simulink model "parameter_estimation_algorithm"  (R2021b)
settings: Solver=FixedStepDiscrete  StartTime=0.0  StopTime=10.0  RelTol=1e-3
InitFcn:
  | parameter_estimation_init;
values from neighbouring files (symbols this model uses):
  ADC_resolution = 12    [parameter_estimation_init.m]
  Ts = 1/PWM_frequency    (= 5e-05)    [parameter_estimation_init.m]
undefined symbols (not defined in the file or in its folder): bits, case, DiscIntNeverNeededParam, inverter
libraries: mcbcontrolslib x14, mcbpositiondecoderlib x3, simulink x2
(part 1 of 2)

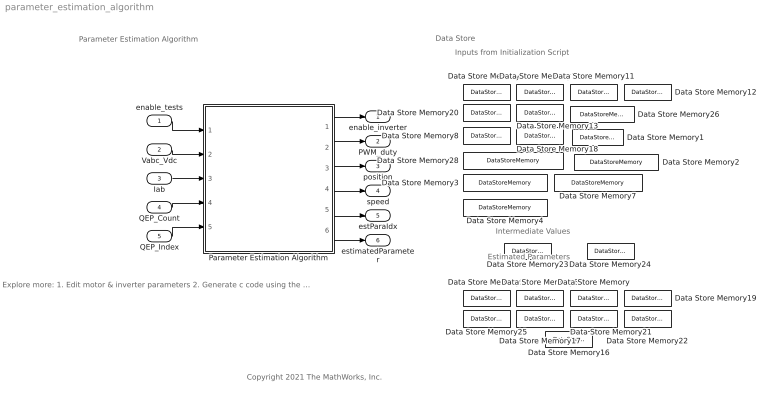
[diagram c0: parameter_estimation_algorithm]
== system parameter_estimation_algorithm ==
  note: Estimated Parameters
  note: Inputs from Initialization Script
  note: Data Store
  note: Intermediate Values
  note: Explore more: 1. Edit motor & inverter parameters 2. Generate c code using the 'Embedded Coder' app 3. Integrate generated code with driver code
  note: Parameter Estimation Algorithm
  note: Copyright 2021 The MathWorks, Inc.
  enable_tests : Inport  OutDataTypeStr=single
  Vabc_Vdc : Inport  Port=2  OutDataTypeStr=uint16
  Iab : Inport  Port=3  OutDataTypeStr=uint16
  QEP_Count : Inport  Port=4  OutDataTypeStr=uint16
  QEP_Index : Inport  Port=5  OutDataTypeStr=uint16
  Data Store Memory : DataStoreMemory  DataStoreName=Rs  ReadBeforeWriteMsg=warning  WriteAfterWriteMsg=warning  WriteAfterReadMsg=warning  ShowAdditionalParam=off  OutDataTypeStr=single
  Data Store Memory1 : DataStoreMemory  DataStoreName=testEnable  ReadBeforeWriteMsg=warning  WriteAfterWriteMsg=warning  WriteAfterReadMsg=warning  ShowAdditionalParam=off  OutDataTypeStr=single
  Data Store Memory10 : DataStoreMemory  DataStoreName=V_rated  ReadBeforeWriteMsg=warning  WriteAfterWriteMsg=warning  WriteAfterReadMsg=warning  InitialValue=motorParam.v_dc  ShowAdditionalParam=off  OutDataTypeStr=single
  Data Store Memory11 : DataStoreMemory  DataStoreName=speed_rated  ReadBeforeWriteMsg=warning  WriteAfterWriteMsg=warning  WriteAfterReadMsg=warning  InitialValue=motorParam.ratedSpeed  ShowAdditionalParam=off  OutDataTypeStr=single
  Data Store Memory12 : DataStoreMemory  DataStoreName=pole_pairs  ReadBeforeWriteMsg=warning  WriteAfterWriteMsg=warning  WriteAfterReadMsg=warning  InitialValue=motorParam.p  ShowAdditionalParam=off  OutDataTypeStr=single
  Data Store Memory13 : DataStoreMemory  DataStoreName=RsMeasTestTime  ReadBeforeWriteMsg=warning  WriteAfterWriteMsg=warning  WriteAfterReadMsg=warning  InitialValue=RsMeasTestTime  ShowAdditionalParam=off  OutDataTypeStr=single
  Data Store Memory16 : DataStoreMemory  DataStoreName=Ld  ReadBeforeWriteMsg=warning  WriteAfterWriteMsg=warning  WriteAfterReadMsg=warning  ShowAdditionalParam=off
  Data Store Memory17 : DataStoreMemory  DataStoreName=Lq  ReadBeforeWriteMsg=warning  WriteAfterWriteMsg=warning  WriteAfterReadMsg=warning  ShowAdditionalParam=off
  Data Store Memory18 : DataStoreMemory  DataStoreName=sigma  ReadBeforeWriteMsg=warning  WriteAfterWriteMsg=warning  WriteAfterReadMsg=warning  InitialValue=Ts * 1e6  ShowAdditionalParam=off  OutDataTypeStr=single
  Data Store Memory19 : DataStoreMemory  DataStoreName=Bemf  ReadBeforeWriteMsg=warning  WriteAfterWriteMsg=warning  WriteAfterReadMsg=warning  ShowAdditionalParam=off
  Data Store Memory2 : DataStoreMemory  DataStoreName=FrequencySweepMax  ReadBeforeWriteMsg=warning  WriteAfterWriteMsg=warning  WriteAfterReadMsg=warning  InitialValue=FrequencySweepMax  ShowAdditionalParam=off  OutDataTypeStr=single
  Data Store Memory20 : DataStoreMemory  DataStoreName=R_board  ReadBeforeWriteMsg=warning  WriteAfterWriteMsg=warning  WriteAfterReadMsg=warning  InitialValue=inverter.R_board  ShowAdditionalParam=off
  Data Store Memory21 : DataStoreMemory  DataStoreName=J  ReadBeforeWriteMsg=warning  WriteAfterWriteMsg=warning  WriteAfterReadMsg=warning  ShowAdditionalParam=off
  Data Store Memory22 : DataStoreMemory  DataStoreName=B  ReadBeforeWriteMsg=warning  WriteAfterWriteMsg=warning  WriteAfterReadMsg=warning  ShowAdditionalParam=off
  Data Store Memory23 : DataStoreMemory  DataStoreName=Kp_i  ReadBeforeWriteMsg=warning  WriteAfterWriteMsg=warning  WriteAfterReadMsg=warning  ShowAdditionalParam=off  OutDataTypeStr=single
  Data Store Memory24 : DataStoreMemory  DataStoreName=Ki_i  ReadBeforeWriteMsg=warning  WriteAfterWriteMsg=warning  WriteAfterReadMsg=warning  ShowAdditionalParam=off  OutDataTypeStr=single
  Data Store Memory25 : DataStoreMemory  DataStoreName=errorID  ReadBeforeWriteMsg=warning  WriteAfterWriteMsg=warning  WriteAfterReadMsg=warning  ShowAdditionalParam=off
  Data Store Memory26 : DataStoreMemory  DataStoreName=Position_offset  ReadBeforeWriteMsg=warning  WriteAfterWriteMsg=warning  WriteAfterReadMsg=warning  InitialValue=motorParam.PositionOffset  ShowAdditionalParam=off  OutDataTypeStr=single
  Data Store Memory28 : DataStoreMemory  DataStoreName=inverter_V_max  ReadBeforeWriteMsg=warning  WriteAfterWriteMsg=warning  WriteAfterReadMsg=warning  InitialValue=inverter.V_max  ShowAdditionalParam=off  OutDataTypeStr=single
  Data Store Memory3 : DataStoreMemory  DataStoreName=FrequencySweepMin  ReadBeforeWriteMsg=warning  WriteAfterWriteMsg=warning  WriteAfterReadMsg=warning  InitialValue=FrequencySweepMin  ShowAdditionalParam=off  OutDataTypeStr=single
  Data Store Memory4 : DataStoreMemory  DataStoreName=FrequencySweepStep  ReadBeforeWriteMsg=warning  WriteAfterWriteMsg=warning  WriteAfterReadMsg=warning  InitialValue=FrequencySweepStep  ShowAdditionalParam=off  OutDataTypeStr=single
  Data Store Memory5 : DataStoreMemory  DataStoreName=Ia_avg_cal  ReadBeforeWriteMsg=warning  WriteAfterWriteMsg=warning  WriteAfterReadMsg=warning  ShowAdditionalParam=off  OutDataTypeStr=single
  Data Store Memory6 : DataStoreMemory  DataStoreName=Ib_avg_cal  ReadBeforeWriteMsg=warning  WriteAfterWriteMsg=warning  WriteAfterReadMsg=warning  ShowAdditionalParam=off  OutDataTypeStr=single
  Data Store Memory7 : DataStoreMemory  DataStoreName=DaxisVoltageReference  ReadBeforeWriteMsg=warning  WriteAfterWriteMsg=warning  WriteAfterReadMsg=warning  InitialValue=DaxisVoltageReference  ShowAdditionalParam=off  OutDataTypeStr=single
  Data Store Memory8 : DataStoreMemory  DataStoreName=currentPU_RWV  ReadBeforeWriteMsg=warning  WriteAfterWriteMsg=warning  WriteAfterReadMsg=warning  InitialValue=inverter.I_max  ShowAdditionalParam=off  OutDataTypeStr=single
  Data Store Memory9 : DataStoreMemory  DataStoreName=I_rated  ReadBeforeWriteMsg=warning  WriteAfterWriteMsg=warning  WriteAfterReadMsg=warning  InitialValue=motorParam.nomCurrent  ShowAdditionalParam=off  OutDataTypeStr=single
  Parameter Estimation Algorithm : Subsystem
  enable_inverter : Outport
  PWM_duty : Outport  Port=2
  position : Outport  Port=3
  speed : Outport  Port=4
  estParaIdx : Outport  Port=5
  estimatedParameter : Outport  Port=6
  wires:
  QEP_Index/1 -> Parameter Estimation Algorithm/5(QEP_Index)
  Parameter Estimation Algorithm/2(PWM_duty) -> PWM_duty/1
  Vabc_Vdc/1 -> Parameter Estimation Algorithm/2(Vabc_Vdc)
  Iab/1 -> Parameter Estimation Algorithm/3(Iab)
  enable_tests/1 -> Parameter Estimation Algorithm/1(enable)
  QEP_Count/1 -> Parameter Estimation Algorithm/4(QEP_Count)
  Parameter Estimation Algorithm/1(enable_inverter) -> enable_inverter/1
  Parameter Estimation Algorithm/3(Position) -> position/1
  Parameter Estimation Algorithm/4(Speed) -> speed/1
  Parameter Estimation Algorithm/5(estParIdx) -> estParaIdx/1
  Parameter Estimation Algorithm/6(estimatedParameter) -> estimatedParameter/1

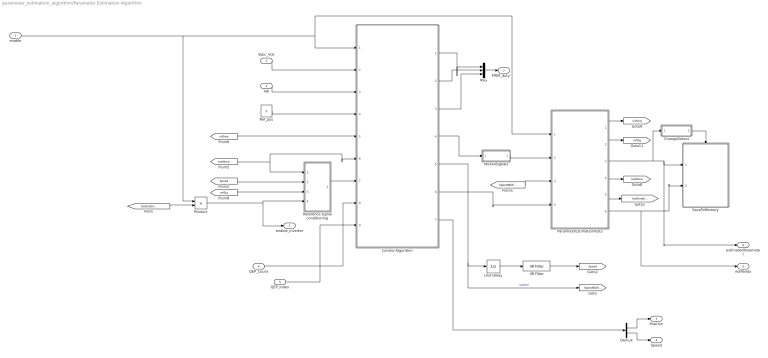
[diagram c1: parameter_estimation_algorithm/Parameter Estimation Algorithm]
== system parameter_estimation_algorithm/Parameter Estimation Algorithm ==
  enable : Inport
  Vabc_Vdc : Inport  Port=2  PortDimensions=4
  Iab : Inport  Port=3  PortDimensions=2
  QEP_Count : Inport  Port=4
  QEP_Index : Inport  Port=5
  ChangeDetect : Subsystem
  Control Algorithm : Subsystem
  Demux : Demux  Outputs=2
  IIR Filter : mcbcontrolslib/IIR Filter  VariantControl=Low Pass Filter  VariantSelect=Low-pass  Filter_constant=0.01  advancedSettings=off  Ts=50e-6  cutOff_freq=32.1525
  Mux : Mux  Inputs=3
  MuxAllSignals : Subsystem
  ParameterEstimationTests : Subsystem
  Product : Product  OutDataTypeStr=single
  Ref_pos : Constant  Value=0  OutDataTypeStr=single  SampleTime=-1
  Reference signal conditioning : Subsystem
  SaveToMemory : Subsystem
  Unit Delay : UnitDelay  SampleTime=-1  HasFrameUpgradeWarning=on
  enable_inverter : Outport
  PWM_duty : Outport  Port=2
  Position : Outport  Port=3
  Speed : Outport  Port=4
  estParIdx : Outport  Port=5
  estimatedParameter : Outport  Port=6
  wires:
  [testNum] -> Reference signal conditioning/1(TestNum), Control Algorithm/6(TestNum)
  [injFreq] -> Control Algorithm/5(Freq)
  Control Algorithm/4(Ia_Ib_ADC_count or VdId or VqIq or VaVb) -> MuxAllSignals/1(Sig)
  [Speed] -> Reference signal conditioning/2(ActSpeed)
  Control Algorithm/5(Speed) -> [SpeedWOfilter], Unit Delay/1  "speed"
  Reference signal conditioning/1(Out2) -> Control Algorithm/7(RefSignal)
  Control Algorithm/6(Vdc) -> ParameterEstimationTests/4(Vdc)
  ParameterEstimationTests/2(refSignalOut) -> [refSig]
  ParameterEstimationTests/1(injFreqOut) -> [injFreq]
  [refSig] -> Reference signal conditioning/3("RefSignal ")
  Product/1 -> enable_inverter/1, Reference signal conditioning/4(Running)
  ParameterEstimationTests/3(estimatedParameter) -> estimatedParameter/1, SaveToMemory/1(estimatedParameter), ChangeDetect/1(Sig)
  ChangeDetect/1(ChangeDet) -> SaveToMemory/Trigger
  ParameterEstimationTests/4(testNumOut) -> [testNum]
  MuxAllSignals/1(AllSig) -> ParameterEstimationTests/2(SignalPU)
  ParameterEstimationTests/6(estParIdx) -> estParIdx/1, SaveToMemory/2(estParIdx)
  ParameterEstimationTests/5(testEnableFromTrgt) -> [testEnableFromTrgt]
  [testEnableFromTrgt] -> Product/2
  Unit Delay/1 -> IIR Filter/1
  IIR Filter/1 -> [Speed]
  [SpeedWOfilter] -> ParameterEstimationTests/3(speed)
  Vabc_Vdc/1 -> Control Algorithm/2(Vabc_Vdc)
  Iab/1 -> Control Algorithm/3(IA/IB)
  Ref_pos/1 -> Control Algorithm/4(Ref_pos)
  Control Algorithm/1(PWM1) -> Mux/1
  Control Algorithm/2(PWM2) -> Mux/2
  Control Algorithm/3(PWM3) -> Mux/3
  QEP_Count/1 -> Control Algorithm/8(QEP_Count)
  QEP_Index/1 -> Control Algorithm/9(QEP_Index)
  enable/1 -> Product/1, ParameterEstimationTests/1(enable), Control Algorithm/1(enable)
  Mux/1 -> PWM_duty/1
  Control Algorithm/7(Pos/Speed) -> Demux/1
  Demux/1 -> Position/1
  Demux/2 -> Speed/1

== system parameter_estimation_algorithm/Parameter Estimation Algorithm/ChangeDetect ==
  Sig : Inport
  Equal : RelationalOperator  Operator=~=  OutDataTypeStr=boolean  RndMeth=Simplest
  Unit Delay : UnitDelay  SampleTime=-1  HasFrameUpgradeWarning=on
  ChangeDet : Outport
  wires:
  Equal/1 -> ChangeDet/1
  Sig/1 -> Equal/2, Unit Delay/1
  Unit Delay/1 -> Equal/1

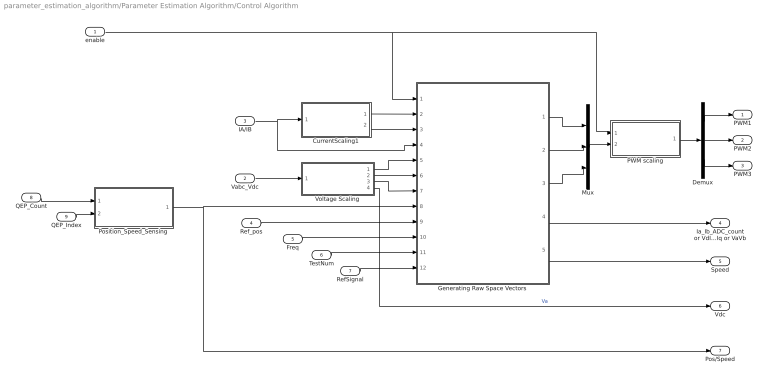
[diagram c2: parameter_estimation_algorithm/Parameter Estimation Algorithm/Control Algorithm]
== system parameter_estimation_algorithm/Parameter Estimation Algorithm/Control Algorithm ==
  enable : Inport
  Vabc_Vdc : Inport  Port=2
  IA/IB : Inport  Port=3
  Ref_pos : Inport  Port=4
  Freq : Inport  Port=5
  TestNum : Inport  Port=6
  RefSignal : Inport  Port=7
  QEP_Count : Inport  Port=8
  QEP_Index : Inport  Port=9
  CurrentScaling1 : Subsystem
  Demux : Demux  Outputs=3
  Generating Raw Space Vectors : Subsystem
  Mux : Mux  Inputs=3
  PWM scaling : Subsystem
  Position_Speed_Sensing : Subsystem
  Voltage Scaling : Subsystem
  PWM1 : Outport  VectorParamsAs1DForOutWhenUnconnected=off
  PWM2 : Outport  Port=2  VectorParamsAs1DForOutWhenUnconnected=off
  PWM3 : Outport  Port=3  VectorParamsAs1DForOutWhenUnconnected=off
  Ia_Ib_ADC_count or VdId or VqIq or VaVb : Outport  Port=4  OutDataTypeStr=single  VectorParamsAs1DForOutWhenUnconnected=off
  Speed : Outport  Port=5  OutDataTypeStr=single  VectorParamsAs1DForOutWhenUnconnected=off
  Vdc : Outport  Port=6  OutDataTypeStr=single  VectorParamsAs1DForOutWhenUnconnected=off
  Pos/Speed : Outport  Port=7
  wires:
  Demux/1 -> PWM1/1
  Demux/3 -> PWM3/1
  Demux/2 -> PWM2/1
  Vabc_Vdc/1 -> Voltage Scaling/1(Vabc)
  IA/IB/1 -> Generating Raw Space Vectors/4(IaIb_adc_counts), CurrentScaling1/1(IA/IB)
  Generating Raw Space Vectors/2(Tb) -> Mux/2
  Voltage Scaling/1(Vao) -> Generating Raw Space Vectors/5(Va0)
  Mux/1 -> PWM scaling/2(Ta/Tb/Tc)
  PWM scaling/1(PWM A/B/C) -> Demux/1
  CurrentScaling1/2(Ib) -> Generating Raw Space Vectors/3(Ib)
  CurrentScaling1/1(Ia) -> Generating Raw Space Vectors/2(Ia)
  Generating Raw Space Vectors/3(Tc) -> Mux/3
  Generating Raw Space Vectors/1(Ta) -> Mux/1
  Ref_pos/1 -> Generating Raw Space Vectors/9(Ref_posOL)
  Freq/1 -> Generating Raw Space Vectors/10(Freq)
  TestNum/1 -> Generating Raw Space Vectors/11(TestNum)
  RefSignal/1 -> Generating Raw Space Vectors/12(RefSignal)
  Generating Raw Space Vectors/4(Ia_Ib_ADC_count or VdId or VqIq or VaVb) -> Ia_Ib_ADC_count or VdId or VqIq or VaVb/1
  Generating Raw Space Vectors/5(Speed) -> Speed/1
  Voltage Scaling/2(Vbo) -> Generating Raw Space Vectors/6(Vb0)
  Voltage Scaling/3(Vco) -> Generating Raw Space Vectors/7(Vco)
  Position_Speed_Sensing/1(Pos/Speed) -> Pos/Speed/1, Generating Raw Space Vectors/8(Pos/Speed)
  Voltage Scaling/4(Vdc) -> Vdc/1  "Va"
  QEP_Count/1 -> Position_Speed_Sensing/1(QEP_Count)
  QEP_Index/1 -> Position_Speed_Sensing/2(QEP_Index)
  enable/1 -> PWM scaling/1(enable), Generating Raw Space Vectors/1(enable)

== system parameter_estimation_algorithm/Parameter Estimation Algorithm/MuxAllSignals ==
  Sig : Inport
  Demux : Demux  Outputs=2
  Demux1 : Demux  Outputs=2
  Demux2 : Demux  Outputs=2
  Mux : Mux  Inputs=6
  AllSig : Outport
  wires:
  Mux/1 -> AllSig/1
  Sig/1 -> Demux/1
  Demux/1 -> Mux/1
  Demux/2 -> Mux/2
  Demux1/2 -> Mux/4
  Demux1/1 -> Mux/3
  Demux2/1 -> Mux/5
  Demux2/2 -> Mux/6
  [VdId_32_Q17] -> Demux1/1
  [VqIq_32_Q17] -> Demux2/1

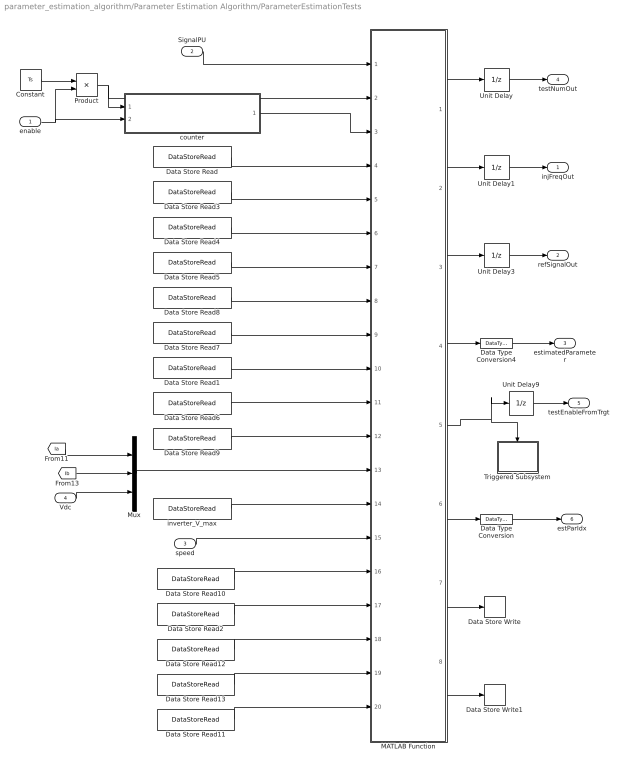
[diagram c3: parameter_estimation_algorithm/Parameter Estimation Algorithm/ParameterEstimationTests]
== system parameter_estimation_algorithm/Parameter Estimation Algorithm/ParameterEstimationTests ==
  enable : Inport
  SignalPU : Inport  Port=2
  speed : Inport  Port=3
  Vdc : Inport  Port=4
  Constant : Constant  Value=Ts  OutDataTypeStr=single  SampleTime=-1
  Data Store Read : DataStoreRead  DataStoreName=RsMeasTestTime  IndexOptions=Index vector (dialog)  Indices=1  OutputSizes=1
  Data Store Read1 : DataStoreRead  DataStoreName=V_rated  IndexOptions=Index vector (dialog)  Indices=1  OutputSizes=1
  Data Store Read10 : DataStoreRead  DataStoreName=speed_rated  IndexOptions=Index vector (dialog)  Indices=1  OutputSizes=1
  Data Store Read11 : DataStoreRead  DataStoreName=FrequencySweepStep  IndexOptions=Index vector (dialog)  Indices=1  OutputSizes=1
  Data Store Read12 : DataStoreRead  DataStoreName=FrequencySweepMin  IndexOptions=Index vector (dialog)  Indices=1  OutputSizes=1
  Data Store Read13 : DataStoreRead  DataStoreName=FrequencySweepMax  IndexOptions=Index vector (dialog)  Indices=1  OutputSizes=1
  Data Store Read2 : DataStoreRead  DataStoreName=DaxisVoltageReference  IndexOptions=Index vector (dialog)  Indices=1  OutputSizes=1
  Data Store Read3 : DataStoreRead  DataStoreName=I_rated  IndexOptions=Index vector (dialog)  Indices=1  OutputSizes=1
  Data Store Read4 : DataStoreRead  DataStoreName=pole_pairs  IndexOptions=Index vector (dialog)  Indices=1  OutputSizes=1
  Data Store Read5 : DataStoreRead  DataStoreName=Rs  IndexOptions=Index vector (dialog)  Indices=1  OutputSizes=1
  Data Store Read6 : DataStoreRead  DataStoreName=currentPU_RWV  IndexOptions=Index vector (dialog)  Indices=1  OutputSizes=1
  Data Store Read7 : DataStoreRead  DataStoreName=R_board  IndexOptions=Index vector (dialog)  Indices=1  OutputSizes=1
  Data Store Read8 : DataStoreRead  DataStoreName=Ld  IndexOptions=Index vector (dialog)  Indices=1  OutputSizes=1
  Data Store Read9 : DataStoreRead  DataStoreName=sigma  IndexOptions=Index vector (dialog)  Indices=1  OutputSizes=1
  Data Store Write : DataStoreWrite  DataStoreName=Kp_i  IndexOptions=Index vector (dialog)  Indices=1  OutputSizes=1
  Data Store Write1 : DataStoreWrite  DataStoreName=Ki_i  IndexOptions=Index vector (dialog)  Indices=1  OutputSizes=1
  Data Type Conversion : DataTypeConversion  OutDataTypeStr=uint32  RndMeth=Simplest
  Data Type Conversion4 : DataTypeConversion  OutDataTypeStr=single  RndMeth=Simplest
  MATLAB Function : MATLAB Function  TreatAsAtomicUnit=on
  Mux : Mux  Inputs=3
  Product : Product  OutDataTypeStr=single
  Triggered Subsystem : Subsystem  TreatAsAtomicUnit=on
  Unit Delay : UnitDelay  SampleTime=-1  HasFrameUpgradeWarning=on
  Unit Delay1 : UnitDelay  SampleTime=-1  HasFrameUpgradeWarning=on
  Unit Delay3 : UnitDelay  SampleTime=-1  HasFrameUpgradeWarning=on
  Unit Delay9 : UnitDelay  InitialCondition=1  SampleTime=-1  HasFrameUpgradeWarning=on
  counter : Subsystem
  inverter_V_max : DataStoreRead  DataStoreName=inverter_V_max  IndexOptions=Index vector (dialog)  Indices=1  OutputSizes=1
  injFreqOut : Outport  InitialOutput=[0]
  refSignalOut : Outport  Port=2  InitialOutput=[0]
  estimatedParameter : Outport  Port=3  InitialOutput=[0]
  testNumOut : Outport  Port=4  InitialOutput=[0]
  testEnableFromTrgt : Outport  Port=5  InitialOutput=[0]
  estParIdx : Outport  Port=6  InitialOutput=[0]
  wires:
  Data Store Read11/1 -> MATLAB Function/20(freqStep)
  Data Store Read13/1 -> MATLAB Function/19(freqMax)
  Data Store Read8/1 -> MATLAB Function/8(Ld)
  Data Store Read12/1 -> MATLAB Function/18(freqMin)
  speed/1 -> MATLAB Function/15(speedFB)
  Data Type Conversion4/1 -> estimatedParameter/1
  [Ia] -> Mux/1
  Data Store Read2/1 -> MATLAB Function/17(Vd_ref_Rs)
  [Ib] -> Mux/2
  Data Store Read10/1 -> MATLAB Function/16(speed_rated)
  SignalPU/1 -> MATLAB Function/1(SignalsPU)
  counter/1(curTime) -> MATLAB Function/3(curTime)
  Data Store Read7/1 -> MATLAB Function/9(R_board)
  Unit Delay3/1 -> refSignalOut/1
  MATLAB Function/7(Kp_iOut) -> Data Store Write/1
  Unit Delay1/1 -> injFreqOut/1
  Unit Delay/1 -> testNumOut/1
  MATLAB Function/3(refSignalOut) -> Unit Delay3/1
  Vdc/1 -> Mux/3
  MATLAB Function/2(injFreqOut) -> Unit Delay1/1
  MATLAB Function/1(testNumOut) -> Unit Delay/1
  inverter_V_max/1 -> MATLAB Function/14(inverter_V_max)
  MATLAB Function/4(estimatedParameterOut) -> Data Type Conversion4/1
  Mux/1 -> MATLAB Function/13(IaIbVdc)
  Data Store Read/1 -> MATLAB Function/4(RsMeasTestTime)
  MATLAB Function/5(testEnableOut) -> Unit Delay9/1, Triggered Subsystem/Trigger
  Constant/1 -> Product/1
  Data Store Read1/1 -> MATLAB Function/10(V_rated)
  Data Store Read3/1 -> MATLAB Function/5(I_rated)
  Data Store Read4/1 -> MATLAB Function/6(pole_pairs)
  Data Store Read5/1 -> MATLAB Function/7(Rs)
  Unit Delay9/1 -> testEnableFromTrgt/1
  Product/1 -> MATLAB Function/2(Ts), counter/1(Ts)
  MATLAB Function/6(estParIdxOut) -> Data Type Conversion/1
  Data Store Read9/1 -> MATLAB Function/12(sigma)
  Data Type Conversion/1 -> estParIdx/1
  Data Store Read6/1 -> MATLAB Function/11(currentPU_RWV)
  MATLAB Function/8(Ki_iOut) -> Data Store Write1/1
  enable/1 -> counter/2(testEnableFromHost), Product/2

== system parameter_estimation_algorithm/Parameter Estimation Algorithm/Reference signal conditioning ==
  TestNum : Inport
  ActSpeed : Inport  Port=2
  "RefSignal " : Inport  Port=3
  Running : Inport  Port=4
  Compare To Constant : simulink/Logic and Bit Operations/Compare To Constant  relop=>=  const=4  OutDataTypeStr=boolean
  Data Type Conversion3 : DataTypeConversion  OutDataTypeStr=single
  Switch : Switch  Threshold=4
  TestNum1 : InportShadow
  Torque_control_with_speed_limit : Subsystem
  Out2 : Outport  VectorParamsAs1DForOutWhenUnconnected=off
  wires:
  Switch/1 -> Data Type Conversion3/1
  TestNum/1 -> Switch/2
  Data Type Conversion3/1 -> Out2/1
  "RefSignal "/1 -> Torque_control_with_speed_limit/1(MaxSpeed), Switch/3
  ActSpeed/1 -> Torque_control_with_speed_limit/2(ActSpeed)
  Running/1 -> Torque_control_with_speed_limit/3(En)
  Torque_control_with_speed_limit/1(Iq_ref) -> Switch/1
  Compare To Constant/1 -> Torque_control_with_speed_limit/Enable
  TestNum1/1 -> Compare To Constant/1

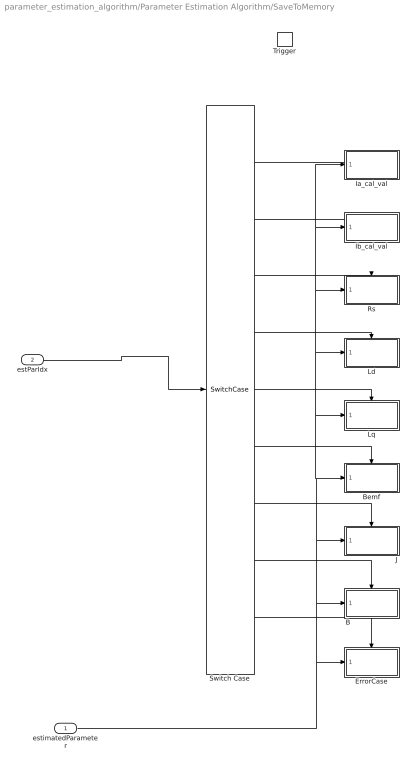
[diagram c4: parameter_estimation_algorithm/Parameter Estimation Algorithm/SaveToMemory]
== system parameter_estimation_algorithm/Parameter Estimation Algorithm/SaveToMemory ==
  estimatedParameter : Inport
  estParIdx : Inport  Port=2
  Trigger : TriggerPort  TriggerType=either  VariantControl=Variant  PortDimensions=1
  B : Subsystem  TreatAsAtomicUnit=on
  Bemf : Subsystem  TreatAsAtomicUnit=on
  ErrorCase : Subsystem  TreatAsAtomicUnit=on
  Ia_cal_val : Subsystem  TreatAsAtomicUnit=on
  Ib_cal_val : Subsystem  TreatAsAtomicUnit=on
  J : Subsystem  TreatAsAtomicUnit=on
  Ld : Subsystem  TreatAsAtomicUnit=on
  Lq : Subsystem  TreatAsAtomicUnit=on
  Rs : Subsystem  TreatAsAtomicUnit=on
  Switch Case : SwitchCase  CaseConditions={0 1 2 3 4 5 6 7 8}  ShowDefaultCase=off
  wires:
  Switch Case/9 -> ErrorCase/Action
  Switch Case/7 -> J/Action
  Switch Case/8 -> B/Action
  Switch Case/6 -> Bemf/Action
  estimatedParameter/1 -> ErrorCase/1(In1), B/1(In1), J/1(In1), Bemf/1(In1), Lq/1(In1), Ld/1(In1), Rs/1(In1), Ib_cal_val/1(In1), Ia_cal_val/1(In1)
  estParIdx/1 -> Switch Case/1
  Switch Case/4 -> Ld/Action
  Switch Case/3 -> Rs/Action
  Switch Case/2 -> Ib_cal_val/Action
  Switch Case/1 -> Ia_cal_val/Action
  Switch Case/5 -> Lq/Action

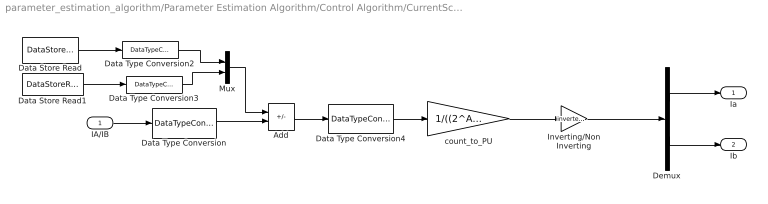
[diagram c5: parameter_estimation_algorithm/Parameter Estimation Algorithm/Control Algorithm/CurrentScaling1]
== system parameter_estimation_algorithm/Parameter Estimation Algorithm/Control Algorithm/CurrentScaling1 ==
  IA/IB : Inport
  Add : Sum  Inputs=-+
  Data Store Read : DataStoreRead  DataStoreName=Ia_avg_cal  IndexOptions=Index vector (dialog)  Indices=1  OutputSizes=1
  Data Store Read1 : DataStoreRead  DataStoreName=Ib_avg_cal  IndexOptions=Index vector (dialog)  Indices=1  OutputSizes=1
  Data Type Conversion : DataTypeConversion  OutDataTypeStr=int32  ConvertRealWorld=Stored Integer (SI)
  Data Type Conversion2 : DataTypeConversion  OutDataTypeStr=int32  RndMeth=Simplest
  Data Type Conversion3 : DataTypeConversion  OutDataTypeStr=int32  RndMeth=Simplest
  Data Type Conversion4 : DataTypeConversion  OutDataTypeStr=single  RndMeth=Simplest
  Demux : Demux  Outputs=2
  Inverting/Non Inverting : Gain  Gain=inverter.invertingAmp  OutDataTypeStr=single
  Mux : Mux  Inputs=2
  count_to_PU : Gain  Gain=1/((2^ADC_resolution)/2)  OutDataTypeStr=single  RndMeth=Simplest
  Ia : Outport  VectorParamsAs1DForOutWhenUnconnected=off
  Ib : Outport  Port=2  VectorParamsAs1DForOutWhenUnconnected=off
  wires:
  IA/IB/1 -> Data Type Conversion/1
  Mux/1 -> Add/1
  Data Type Conversion/1 -> Add/2
  Demux/2 -> Ib/1
  Demux/1 -> Ia/1
  count_to_PU/1 -> Inverting/Non Inverting/1
  Data Store Read1/1 -> Data Type Conversion3/1
  Data Store Read/1 -> Data Type Conversion2/1
  Data Type Conversion2/1 -> Mux/1
  Data Type Conversion3/1 -> Mux/2
  Data Type Conversion4/1 -> count_to_PU/1
  Add/1 -> Data Type Conversion4/1
  Inverting/Non Inverting/1 -> Demux/1

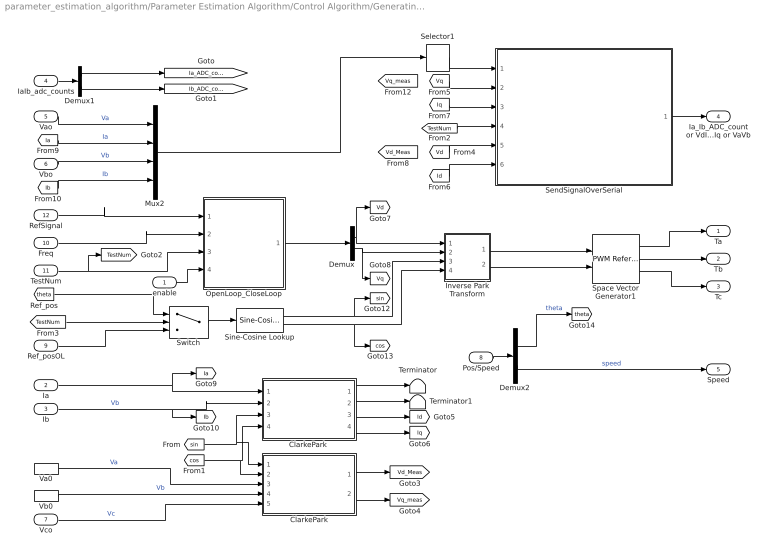
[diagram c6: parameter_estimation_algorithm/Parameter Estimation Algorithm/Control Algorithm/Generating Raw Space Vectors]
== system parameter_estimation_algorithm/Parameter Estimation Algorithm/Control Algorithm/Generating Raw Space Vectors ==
  enable : Inport
  Ia : Inport  Port=2
  Ib : Inport  Port=3
  IaIb_adc_counts : Inport  Port=4
  Vao : Inport  Port=5
  Vbo : Inport  Port=6
  Vco : Inport  Port=7
  Pos/Speed : Inport  Port=8
  Ref_posOL : Inport  Port=9
  Freq : Inport  Port=10
  TestNum : Inport  Port=11
  RefSignal : Inport  Port=12
  ClarkePark : Subsystem
  "ClarkePark " : Subsystem
  Demux : Demux  Outputs=2
  Demux1 : Demux  Outputs=2
  Demux2 : Demux  Outputs=2
  Inverse Park Transform : Subsystem
  Mux2 : Mux
  OpenLoop_CloseLoop : Subsystem
  Selector1 : Selector  InputPortWidth=4  IndexOptions=Index vector (dialog)  Indices=[1 3]  OutputSizes=1
  SendSignalOverSerial : Subsystem
  Sine-Cosine Lookup : mcbcontrolslib/Sine-Cosine Lookup  AngleInput=Per-unit  N_points=1024
  Space Vector Generator1 : mcbcontrolslib/PWM Reference Generator  inSignal=Valphabeta  modType=SVM: space vector modulation
  Switch : Switch  Threshold=4
  Terminator : Terminator
  Terminator1 : Terminator
  Va0 : InportShadow  Port=5
  Vb0 : InportShadow  Port=6
  Ta : Outport  VectorParamsAs1DForOutWhenUnconnected=off
  Tb : Outport  Port=2  VectorParamsAs1DForOutWhenUnconnected=off
  Tc : Outport  Port=3  VectorParamsAs1DForOutWhenUnconnected=off
  Ia_Ib_ADC_count or VdId or VqIq or VaVb : Outport  Port=4  VectorParamsAs1DForOutWhenUnconnected=off
  Speed : Outport  Port=5  VectorParamsAs1DForOutWhenUnconnected=off
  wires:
  Space Vector Generator1/1 -> Ta/1
  Space Vector Generator1/2 -> Tb/1
  Space Vector Generator1/3 -> Tc/1
  Demux/2 -> [Vq], Inverse Park Transform/2(Q)
  Demux/1 -> [Vd], Inverse Park Transform/1(D)
  Freq/1 -> OpenLoop_CloseLoop/2(Freq)
  TestNum/1 -> OpenLoop_CloseLoop/3(TestNum), [TestNum]
  Ia/1 -> "ClarkePark "/1(Ia), [Ia]
  Ib/1 -> "ClarkePark "/2(Ib), [Ib]  "Vb"
  Demux2/1 -> [theta]  "theta"
  RefSignal/1 -> OpenLoop_CloseLoop/1(RefSignal)
  OpenLoop_CloseLoop/1(VdVq) -> Demux/1
  Ref_posOL/1 -> Switch/3
  [TestNum] -> Switch/2
  Pos/Speed/1 -> Demux2/1
  Demux2/2 -> Speed/1  "speed"
  ClarkePark/1(Vd_Meas) -> [Vd_Meas]
  ClarkePark/2(Vq_Meas) -> [Vq_meas]
  Vb0/1 -> ClarkePark/4(Vbo)  "Vb"
  Va0/1 -> ClarkePark/3(Vao)  "Va"
  Vco/1 -> ClarkePark/5(Vco)  "Vc"
  "ClarkePark "/3(D) -> [Id]
  "ClarkePark "/4(Q) -> [Iq]
  [Iq] -> SendSignalOverSerial/3(Iq)
  [TestNum] -> SendSignalOverSerial/4(TestNum)
  [Id] -> SendSignalOverSerial/6(Id)
  SendSignalOverSerial/1(Ia_Ib_ADC_count or VdId or VqIq or VaVb) -> Ia_Ib_ADC_count or VdId or VqIq or VaVb/1
  Vao/1 -> Mux2/1  "Va"
  [Ia] -> Mux2/2  "Ia"
  Vbo/1 -> Mux2/3  "Vb"
  [Ib] -> Mux2/4  "Ib"
  Mux2/1 -> Selector1/1
  Inverse Park Transform/1(Alpha) -> Space Vector Generator1/1
  Inverse Park Transform/2(Beta) -> Space Vector Generator1/2
  Demux1/2 -> [Ib_ADC_counts]
  IaIb_adc_counts/1 -> Demux1/1
  Demux1/1 -> [Ia_ADC_counts]
  Selector1/1 -> SendSignalOverSerial/1(VaVb_Uint16)
  "ClarkePark "/2(Beta) -> Terminator1/1
  "ClarkePark "/1(Alpha) -> Terminator/1
  Switch/1 -> Sine-Cosine Lookup/1
  Sine-Cosine Lookup/1 -> [sin], Inverse Park Transform/3(sin)
  Sine-Cosine Lookup/2 -> [cos], Inverse Park Transform/4(cos)
  [theta] -> Switch/1
  [sin] -> ClarkePark/1(sin), "ClarkePark "/3(sin)
  [cos] -> ClarkePark/2(cos), "ClarkePark "/4(cos)
  [Vq] -> SendSignalOverSerial/2(Vq)
  [Vd] -> SendSignalOverSerial/5(Vd)
  enable/1 -> OpenLoop_CloseLoop/4(enable)

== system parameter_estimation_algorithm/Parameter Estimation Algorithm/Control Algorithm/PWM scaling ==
  enable : Inport
  Ta/Tb/Tc : Inport  Port=2
  Add : Sum
  Constant : Constant  OutDataTypeStr=single
  PWM_Counter_Period : Gain  Gain=0.5  ParamDataTypeStr=single  OutDataTypeStr=single  RndMeth=Simplest
  Product : Product  RndMeth=Simplest
  PWM A/B/C : Outport  VectorParamsAs1DForOutWhenUnconnected=off
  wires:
  Constant/1 -> Add/1
  Ta/Tb/Tc/1 -> Add/2
  Add/1 -> PWM_Counter_Period/1
  PWM_Counter_Period/1 -> Product/1
  enable/1 -> Product/2
  Product/1 -> PWM A/B/C/1

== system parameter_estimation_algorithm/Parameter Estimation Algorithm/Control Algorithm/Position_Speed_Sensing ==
  QEP_Count : Inport
  QEP_Index : Inport  Port=2
  " Calculate Position and Speed" : Subsystem
  Data Store Read6 : DataStoreRead  DataStoreName=Position_offset  IndexOptions=Index vector (dialog)  Indices=1  OutputSizes=1
  Mux2 : Mux  Inputs=2
  Pos/Speed : Outport  VectorParamsAs1DForOutWhenUnconnected=off
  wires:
  Mux2/1 -> Pos/Speed/1
  QEP_Index/1 -> " Calculate Position and Speed"/2(QEP_Index_Latch)
  Data Store Read6/1 -> " Calculate Position and Speed"/3(Offset)
  " Calculate Position and Speed"/1(Theta_e) -> Mux2/1
  " Calculate Position and Speed"/2(speed) -> Mux2/2
  QEP_Count/1 -> " Calculate Position and Speed"/1(QEP_Position_Count)

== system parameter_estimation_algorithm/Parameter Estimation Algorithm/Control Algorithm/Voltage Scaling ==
  Vabc : Inport
  Data Type Conversion4 : DataTypeConversion  OutDataTypeStr=single  RndMeth=Simplest
  Demux : Demux
  count_to_PU : Gain  Gain=1/(2^ADC_resolution)  OutDataTypeStr=single  RndMeth=Simplest
  Vao : Outport  VectorParamsAs1DForOutWhenUnconnected=off
  Vbo : Outport  Port=2  VectorParamsAs1DForOutWhenUnconnected=off
  Vco : Outport  Port=3  VectorParamsAs1DForOutWhenUnconnected=off
  Vdc : Outport  Port=4  VectorParamsAs1DForOutWhenUnconnected=off
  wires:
  Demux/3 -> Vco/1
  count_to_PU/1 -> Demux/1
  Demux/1 -> Vao/1
  Demux/2 -> Vbo/1
  Vabc/1 -> Data Type Conversion4/1
  Demux/4 -> Vdc/1
  Data Type Conversion4/1 -> count_to_PU/1

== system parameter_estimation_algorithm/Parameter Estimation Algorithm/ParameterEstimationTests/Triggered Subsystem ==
  Trigger : TriggerPort  VariantControl=Variant
  Constant : Constant  Value=0  OutDataTypeStr=single  SampleTime=-1
  Data Store Write : DataStoreWrite  DataStoreName=testEnable  IndexOptions=Index vector (dialog)  Indices=1  OutputSizes=1
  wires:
  Constant/1 -> Data Store Write/1

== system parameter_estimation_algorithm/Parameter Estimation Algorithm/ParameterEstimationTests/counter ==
  Ts : Inport
  testEnableFromHost : Inport  Port=2
  Sum : Sum  Inputs=|++  RndMeth=Simplest
  Switch : Switch  Criteria=u2 > Threshold
  Unit Delay8 : UnitDelay  SampleTime=-1  HasFrameUpgradeWarning=on
  curTime : Outport
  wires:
  Ts/1 -> Sum/1
  Sum/1 -> curTime/1, Unit Delay8/1  "curTime"
  Unit Delay8/1 -> Switch/1
  Switch/1 -> Sum/2
  testEnableFromHost/1 -> Switch/2, Switch/3

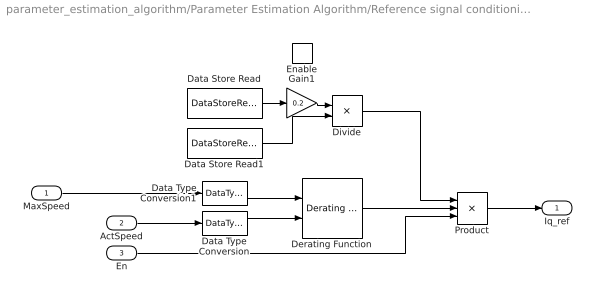
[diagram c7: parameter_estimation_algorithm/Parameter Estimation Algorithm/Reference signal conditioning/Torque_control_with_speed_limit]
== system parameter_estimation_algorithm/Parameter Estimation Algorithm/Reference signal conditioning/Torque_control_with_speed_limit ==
  MaxSpeed : Inport
  ActSpeed : Inport  Port=2
  En : Inport  Port=3
  Enable : EnablePort
  Data Store Read : DataStoreRead  DataStoreName=I_rated  IndexOptions=Index vector (dialog)  Indices=1  OutputSizes=1
  Data Store Read1 : DataStoreRead  DataStoreName=currentPU_RWV  IndexOptions=Index vector (dialog)  Indices=1  OutputSizes=1
  Data Type Conversion : DataTypeConversion  OutDataTypeStr=single
  Data Type Conversion1 : DataTypeConversion  OutDataTypeStr=single
  Derating Function : mcbcontrolslib/Derating Function  x=0.9
  Divide : Product  Inputs=*/  RndMeth=Simplest
  Gain1 : Gain  Gain=0.2  RndMeth=Simplest
  Product : Product  Inputs=3
  Iq_ref : Outport
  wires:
  Gain1/1 -> Divide/1
  Derating Function/1 -> Product/2
  Data Store Read/1 -> Gain1/1
  Data Type Conversion/1 -> Derating Function/2
  Divide/1 -> Product/1
  Product/1 -> Iq_ref/1
  Data Store Read1/1 -> Divide/2
  Data Type Conversion1/1 -> Derating Function/1
  ActSpeed/1 -> Data Type Conversion/1
  MaxSpeed/1 -> Data Type Conversion1/1
  En/1 -> Product/3

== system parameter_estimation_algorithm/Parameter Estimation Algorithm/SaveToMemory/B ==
  In1 : Inport
  Action Port : ActionPort  ActionPortLabel=case [ 7 ]:
  Data Store Write3 : DataStoreWrite  DataStoreName=B  IndexOptions=Index vector (dialog)  Indices=1  OutputSizes=1
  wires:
  In1/1 -> Data Store Write3/1

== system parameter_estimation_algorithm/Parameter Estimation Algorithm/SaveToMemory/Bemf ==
  In1 : Inport
  Action Port : ActionPort  ActionPortLabel=case [ 5 ]:
  Data Store Write3 : DataStoreWrite  DataStoreName=Bemf  IndexOptions=Index vector (dialog)  Indices=1  OutputSizes=1
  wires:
  In1/1 -> Data Store Write3/1

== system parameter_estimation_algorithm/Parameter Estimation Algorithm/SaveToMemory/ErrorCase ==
  In1 : Inport
  Action Port : ActionPort  ActionPortLabel=case [ 8 ]:
  Data Store Write3 : DataStoreWrite  DataStoreName=errorID  IndexOptions=Index vector (dialog)  Indices=1  OutputSizes=1
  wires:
  In1/1 -> Data Store Write3/1

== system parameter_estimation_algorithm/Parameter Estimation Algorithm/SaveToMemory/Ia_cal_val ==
  In1 : Inport
  Action Port : ActionPort  ActionPortLabel=case [ 0 ]:
  Data Store Write1 : DataStoreWrite  DataStoreName=Ia_avg_cal  IndexOptions=Index vector (dialog)  Indices=1  OutputSizes=1
  Gain : Gain  Gain=1e4  RndMeth=Simplest
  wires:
  In1/1 -> Gain/1
  Gain/1 -> Data Store Write1/1

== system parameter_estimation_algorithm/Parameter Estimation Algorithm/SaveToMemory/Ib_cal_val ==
  In1 : Inport
  Action Port : ActionPort  ActionPortLabel=case [ 1 ]:
  Data Store Write2 : DataStoreWrite  DataStoreName=Ib_avg_cal  IndexOptions=Index vector (dialog)  Indices=1  OutputSizes=1
  Gain : Gain  Gain=1e4  RndMeth=Simplest
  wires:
  In1/1 -> Gain/1
  Gain/1 -> Data Store Write2/1

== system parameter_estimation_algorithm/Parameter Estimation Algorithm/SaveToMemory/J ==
  In1 : Inport
  Action Port : ActionPort  ActionPortLabel=case [ 6 ]:
  Data Store Write3 : DataStoreWrite  DataStoreName=J  IndexOptions=Index vector (dialog)  Indices=1  OutputSizes=1
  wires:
  In1/1 -> Data Store Write3/1

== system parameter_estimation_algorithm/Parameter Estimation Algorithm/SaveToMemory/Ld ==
  In1 : Inport
  Action Port : ActionPort  ActionPortLabel=case [ 3 ]:
  Data Store Write4 : DataStoreWrite  DataStoreName=Ld  IndexOptions=Index vector (dialog)  Indices=1  OutputSizes=1
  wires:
  In1/1 -> Data Store Write4/1

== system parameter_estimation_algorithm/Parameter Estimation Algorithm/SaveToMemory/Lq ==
  In1 : Inport
  Action Port : ActionPort  ActionPortLabel=case [ 4 ]:
  Data Store Write3 : DataStoreWrite  DataStoreName=Lq  IndexOptions=Index vector (dialog)  Indices=1  OutputSizes=1
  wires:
  In1/1 -> Data Store Write3/1

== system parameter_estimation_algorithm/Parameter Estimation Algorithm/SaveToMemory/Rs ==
  In1 : Inport
  Action Port : ActionPort  ActionPortLabel=case [ 2 ]:
  Data Store Write2 : DataStoreWrite  DataStoreName=Rs  IndexOptions=Index vector (dialog)  Indices=1  OutputSizes=1
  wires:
  In1/1 -> Data Store Write2/1

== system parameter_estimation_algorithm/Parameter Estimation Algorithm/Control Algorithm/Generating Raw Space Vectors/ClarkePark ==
  sin : Inport
  cos : Inport  Port=2
  Vao : Inport  Port=3
  Vbo : Inport  Port=4
  Vco : Inport  Port=5
  Clarke Transform : mcbcontrolslib/Clarke Transform  VariantControl=Variant2
  Park Transform : mcbcontrolslib/Park Transform  AxisAlignment=D-axis
  Pole_Voltage to Phase_Voltage : Subsystem
  Vd_Meas : Outport  VectorParamsAs1DForOutWhenUnconnected=off
  Vq_Meas : Outport  Port=2  VectorParamsAs1DForOutWhenUnconnected=off
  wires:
  Vco/1 -> Pole_Voltage to Phase_Voltage/3(Vco)
  Clarke Transform/2 -> Park Transform/2
  Pole_Voltage to Phase_Voltage/1(Va) -> Clarke Transform/1
  Park Transform/2 -> Vq_Meas/1  "Vq"
  Clarke Transform/1 -> Park Transform/1
  Pole_Voltage to Phase_Voltage/2(Vb) -> Clarke Transform/2
  Park Transform/1 -> Vd_Meas/1  "Vd"
  Vbo/1 -> Pole_Voltage to Phase_Voltage/2(Vbo)
  Vao/1 -> Pole_Voltage to Phase_Voltage/1(Vao)
  sin/1 -> Park Transform/3
  cos/1 -> Park Transform/4

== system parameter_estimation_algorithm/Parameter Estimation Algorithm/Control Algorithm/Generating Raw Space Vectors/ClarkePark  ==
  Ia : Inport
  Ib : Inport  Port=2
  sin : Inport  Port=3
  cos : Inport  Port=4
  Clarke Transform : mcbcontrolslib/Clarke Transform  VariantControl=Variant2
  Park Transform : mcbcontrolslib/Park Transform  AxisAlignment=D-axis
  Alpha : Outport  VectorParamsAs1DForOutWhenUnconnected=off
  Beta : Outport  Port=2  VectorParamsAs1DForOutWhenUnconnected=off
  D : Outport  Port=3  VectorParamsAs1DForOutWhenUnconnected=off
  Q : Outport  Port=4  VectorParamsAs1DForOutWhenUnconnected=off
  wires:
  Clarke Transform/1 -> Park Transform/1, Alpha/1
  Park Transform/1 -> D/1  "Va"
  Clarke Transform/2 -> Park Transform/2, Beta/1
  Park Transform/2 -> Q/1
  Ib/1 -> Clarke Transform/2
  Ia/1 -> Clarke Transform/1
  sin/1 -> Park Transform/3
  cos/1 -> Park Transform/4

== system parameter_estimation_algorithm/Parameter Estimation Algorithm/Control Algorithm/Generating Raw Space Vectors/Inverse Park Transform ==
  D : Inport
  Q : Inport  Port=2
  sin : Inport  Port=3
  cos : Inport  Port=4
  Inverse Park Transform : mcbcontrolslib/Inverse Park Transform  AxisAlignment=D-axis
  Alpha : Outport  VectorParamsAs1DForOutWhenUnconnected=off
  Beta : Outport  Port=2  VectorParamsAs1DForOutWhenUnconnected=off
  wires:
  Inverse Park Transform/2 -> Beta/1
  sin/1 -> Inverse Park Transform/3
  Q/1 -> Inverse Park Transform/2
  cos/1 -> Inverse Park Transform/4
  Inverse Park Transform/1 -> Alpha/1
  D/1 -> Inverse Park Transform/1

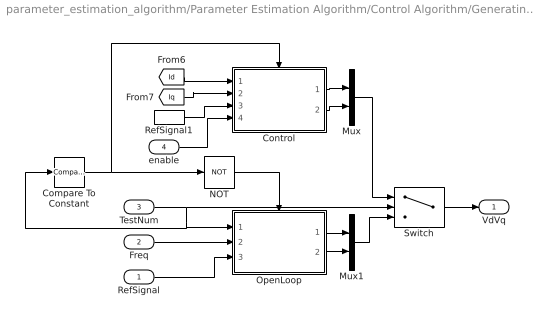
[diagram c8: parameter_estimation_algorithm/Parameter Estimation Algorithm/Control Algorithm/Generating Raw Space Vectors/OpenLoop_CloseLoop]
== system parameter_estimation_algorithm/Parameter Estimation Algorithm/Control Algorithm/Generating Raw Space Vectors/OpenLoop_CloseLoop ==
  RefSignal : Inport
  Freq : Inport  Port=2
  TestNum : Inport  Port=3
  enable : Inport  Port=4
  Compare To Constant : simulink/Logic and Bit Operations/Compare To Constant  relop=>=  const=4  OutDataTypeStr=boolean
  Control : Subsystem
  Mux : Mux  Inputs=2
  Mux1 : Mux  Inputs=2
  NOT : Logic  Operator=NOT  IconShape=distinctive  AllPortsSameDT=off  OutDataTypeStr=boolean
  OpenLoop : Subsystem
  RefSignal1 : InportShadow
  Switch : Switch  Threshold=4
  VdVq : Outport  VectorParamsAs1DForOutWhenUnconnected=off
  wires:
  Freq/1 -> OpenLoop/2(Freq)
  TestNum/1 -> OpenLoop/1(TestNum), Compare To Constant/1, Switch/2
  [Iq] -> Control/2(Iq)
  [Id] -> Control/1(Id)
  Control/1(Vd) -> Mux/1
  Control/2(Vq) -> Mux/2
  OpenLoop/1(RefVd) -> Mux1/1
  OpenLoop/2(RefVq) -> Mux1/2
  Mux/1 -> Switch/1
  Mux1/1 -> Switch/3
  Switch/1 -> VdVq/1
  Compare To Constant/1 -> Control/Enable, NOT/1
  NOT/1 -> OpenLoop/Enable
  RefSignal/1 -> OpenLoop/3(RefSignal)
  RefSignal1/1 -> Control/3(Iq desired)
  enable/1 -> Control/4(enable)

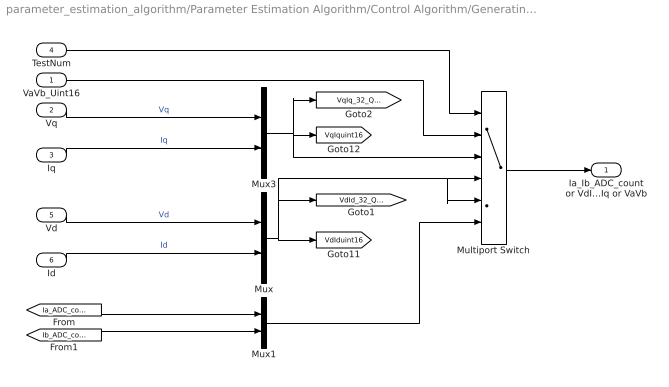
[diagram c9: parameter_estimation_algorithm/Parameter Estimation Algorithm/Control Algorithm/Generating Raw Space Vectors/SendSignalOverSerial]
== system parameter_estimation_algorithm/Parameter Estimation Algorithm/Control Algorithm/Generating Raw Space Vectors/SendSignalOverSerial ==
  VaVb_Uint16 : Inport
  Vq : Inport  Port=2
  Iq : Inport  Port=3
  TestNum : Inport  Port=4
  Vd : Inport  Port=5
  Id : Inport  Port=6
  Multiport Switch : MultiPortSwitch  DataPortOrder=Specify indices  Inputs=2  DataPortIndices={4,3,2,1,0}  OutDataTypeStr=single  RndMeth=Simplest
  Mux : Mux  Inputs=2
  Mux1 : Mux  Inputs=2
  Mux3 : Mux  Inputs=2
  Ia_Ib_ADC_count or VdId or VqIq or VaVb : Outport  OutDataTypeStr=single  VectorParamsAs1DForOutWhenUnconnected=off
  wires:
  Mux/1 -> [VdIduint16], Multiport Switch/5, Multiport Switch/4, [VdId_32_Q17]
  Iq/1 -> Mux3/2  "Iq"
  Vq/1 -> Mux3/1  "Vq"
  Vd/1 -> Mux/1  "Vd"
  TestNum/1 -> Multiport Switch/1
  Mux3/1 -> [VqIq_32_Q17], [VqIquint16], Multiport Switch/3
  Id/1 -> Mux/2  "Id"
  Multiport Switch/1 -> Ia_Ib_ADC_count or VdId or VqIq or VaVb/1
  VaVb_Uint16/1 -> Multiport Switch/2
  Mux1/1 -> Multiport Switch/6
  [Ia_ADC_counts] -> Mux1/1
  [Ib_ADC_counts] -> Mux1/2

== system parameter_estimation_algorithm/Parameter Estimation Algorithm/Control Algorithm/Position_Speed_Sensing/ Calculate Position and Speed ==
  QEP_Position_Count : Inport
  QEP_Index_Latch : Inport  Port=2
  Offset : Inport  Port=3
  IIR Filter : mcbcontrolslib/IIR Filter  VariantControl=Low Pass Filter  VariantSelect=Low-pass  Filter_constant=0.01  advancedSettings=off  Ts=50e-6  cutOff_freq=32.1525
  Mechanical to Electrical Position : mcbpositiondecoderlib/Mechanical to Electrical Position  NrPP=motorParam.p  selectedRange=Per unit  MechOfstInputType=Input port  mechOffsetIn=0  maxAngleIn=1  InputDataType=single  VariantSelect=floating-point
  Quadrature Decoder : mcbpositiondecoderlib/Quadrature Decoder  EncoderSlitsPerRevolution=motorParam.QEPSlits  EncoderCountsPerSlit=4  CounterSize=16 bits  ExternalIndexCount=on  PositionUnit=Per unit  PositionDataType=single
  Speed Measurement : mcbpositiondecoderlib/Speed Measurement  PositionUnit=Per unit  PositionScalingDatatype=uint32  SpeedCalculationMode=Time interval for speed calculation  SampleTimeAsync=Ts  MaximumApplicationSpeed=6000  SpeedResolution=5e-6  DelayLength=20  MaximumMeasurableSpeed=29999  MeasurableSpeedResolution=1.397e-05  SpeedUnit=Per unit based on dialog  PerUnitSpeed=motorParam.ratedSpeed  SpeedDataType=single
  Theta_e : Outport  VectorParamsAs1DForOutWhenUnconnected=off
  speed : Outport  Port=2  VectorParamsAs1DForOutWhenUnconnected=off
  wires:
  Mechanical to Electrical Position/1 -> Theta_e/1
  Speed Measurement/1 -> IIR Filter/1
  Quadrature Decoder/1 -> Mechanical to Electrical Position/1, Speed Measurement/1
  QEP_Position_Count/1 -> Quadrature Decoder/1
  Offset/1 -> Mechanical to Electrical Position/2
  IIR Filter/1 -> speed/1
  QEP_Index_Latch/1 -> Quadrature Decoder/2

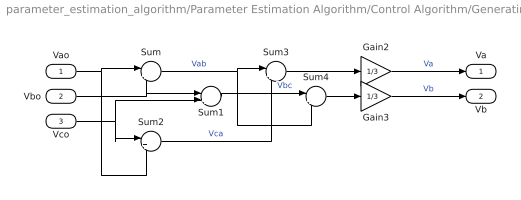
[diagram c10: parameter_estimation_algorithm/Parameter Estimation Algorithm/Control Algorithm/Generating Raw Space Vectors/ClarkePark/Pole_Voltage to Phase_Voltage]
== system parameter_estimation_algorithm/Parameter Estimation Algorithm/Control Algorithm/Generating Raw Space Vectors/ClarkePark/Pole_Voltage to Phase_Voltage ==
  Vao : Inport
  Vbo : Inport  Port=2
  Vco : Inport  Port=3
  Gain2 : Gain  Gain=1/3  RndMeth=Simplest
  Gain3 : Gain  Gain=1/3  RndMeth=Simplest
  Sum{,1..4} (5 alike) : Sum  Inputs=|+-
  Va : Outport  VectorParamsAs1DForOutWhenUnconnected=off
  Vb : Outport  Port=2  VectorParamsAs1DForOutWhenUnconnected=off
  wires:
  Sum1/1 -> Sum4/1  "Vbc"
  Sum2/1 -> Sum3/2  "Vca"
  Sum3/1 -> Gain2/1
  Gain3/1 -> Vb/1  "Vb"
  Sum/1 -> Sum3/1, Sum4/2  "Vab"
  Vco/1 -> Sum1/2, Sum2/1
  Sum4/1 -> Gain3/1
  Gain2/1 -> Va/1  "Va"
  Vbo/1 -> Sum/2, Sum1/1
  Vao/1 -> Sum/1, Sum2/2

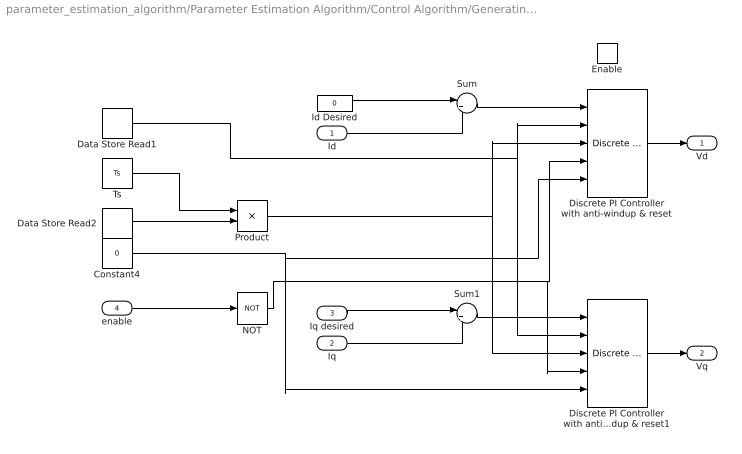
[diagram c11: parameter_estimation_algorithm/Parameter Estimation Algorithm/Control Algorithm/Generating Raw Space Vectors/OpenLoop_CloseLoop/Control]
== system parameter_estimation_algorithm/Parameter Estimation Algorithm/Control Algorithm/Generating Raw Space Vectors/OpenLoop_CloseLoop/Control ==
  Id : Inport
  Iq : Inport  Port=2
  Iq desired : Inport  Port=3
  enable : Inport  Port=4
  Enable : EnablePort
  Constant4 : Constant  Value=0  OutDataTypeStr=single  SampleTime=-1
  Data Store Read1 : DataStoreRead  DataStoreName=Kp_i  IndexOptions=Index vector (dialog)  Indices=1  OutputSizes=1
  Data Store Read2 : DataStoreRead  DataStoreName=Ki_i  IndexOptions=Index vector (dialog)  Indices=1  OutputSizes=1
  Discrete PI Controller with anti-windup & reset : mcbcontrolslib/Discrete PI Controller  with anti-windup & reset  UpperSaturationLimit=0.707  LowerSaturationLimit=-0.707
  Discrete PI Controller with anti-windup & reset1 : mcbcontrolslib/Discrete PI Controller  with anti-windup & reset  UpperSaturationLimit=0.707  LowerSaturationLimit=-0.707
  Id Desired : Constant  Value=0  OutDataTypeStr=single
  NOT : Logic  Operator=NOT  AllPortsSameDT=off  OutDataTypeStr=boolean
  Product : Product
  Sum : Sum  Inputs=|+-
  Sum1 : Sum  Inputs=|+-
  Ts : Constant  Value=Ts  OutDataTypeStr=single  SampleTime=-1
  Vd : Outport  VectorParamsAs1DForOutWhenUnconnected=off
  Vq : Outport  Port=2  VectorParamsAs1DForOutWhenUnconnected=off
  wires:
  Id/1 -> Sum/2
  Iq/1 -> Sum1/2
  Iq desired/1 -> Sum1/1
  Discrete PI Controller with anti-windup & reset/1 -> Vd/1
  Discrete PI Controller with anti-windup & reset1/1 -> Vq/1
  Id Desired/1 -> Sum/1
  Sum1/1 -> Discrete PI Controller with anti-windup & reset1/1
  Sum/1 -> Discrete PI Controller with anti-windup & reset/1
  Product/1 -> Discrete PI Controller with anti-windup & reset1/3, Discrete PI Controller with anti-windup & reset/3
  Constant4/1 -> Discrete PI Controller with anti-windup & reset/5, Discrete PI Controller with anti-windup & reset1/5
  enable/1 -> NOT/1
  NOT/1 -> Discrete PI Controller with anti-windup & reset1/4, Discrete PI Controller with anti-windup & reset/4
  Data Store Read1/1 -> Discrete PI Controller with anti-windup & reset1/2, Discrete PI Controller with anti-windup & reset/2
  Ts/1 -> Product/1
  Data Store Read2/1 -> Product/2

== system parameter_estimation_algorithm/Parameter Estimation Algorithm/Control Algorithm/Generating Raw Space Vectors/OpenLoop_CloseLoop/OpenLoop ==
  TestNum : Inport
  Freq : Inport  Port=2
  RefSignal : Inport  Port=3
  Enable : EnablePort
  ADC_Calibration : Subsystem
  BiasedSineWaveLdMeas : Subsystem
  Demux : Demux  Outputs=2
  Index Vector : MultiPortSwitch  DataPortOrder=Zero-based contiguous  Inputs=4  zeroidx=on
  Rs_Measurement : Subsystem
  SineWaveLqMeas : Subsystem
  RefVd : Outport  VectorParamsAs1DForOutWhenUnconnected=off
  RefVq : Outport  Port=2  VectorParamsAs1DForOutWhenUnconnected=off
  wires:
  Demux/1 -> RefVd/1
  Demux/2 -> RefVq/1
  BiasedSineWaveLdMeas/1(RefVdVq) -> Index Vector/4
  Freq/1 -> BiasedSineWaveLdMeas/2(Freq), SineWaveLqMeas/2(Freq)
  TestNum/1 -> Index Vector/1
  Index Vector/1 -> Demux/1
  Rs_Measurement/1(RefVdVq) -> Index Vector/3  "Rs_Measurement:1"
  ADC_Calibration/1(RefVdVq) -> Index Vector/2  "ADC_Calibration:1"
  RefSignal/1 -> Rs_Measurement/1(Vd_ref), BiasedSineWaveLdMeas/1(Vd_ref), SineWaveLqMeas/1(Vd_ref)
  SineWaveLqMeas/1(RefVdVq) -> Index Vector/5

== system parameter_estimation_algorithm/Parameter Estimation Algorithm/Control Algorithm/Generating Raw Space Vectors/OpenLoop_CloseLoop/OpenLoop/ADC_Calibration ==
  Constant1 : Constant  Value=0  OutDataTypeStr=single  SampleTime=-1
  Constant2 : Constant  Value=0  OutDataTypeStr=single  SampleTime=-1
  Mux : Mux  Inputs=2
  RefVdVq : Outport  VectorParamsAs1DForOutWhenUnconnected=off
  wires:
  Constant2/1 -> Mux/2
  Constant1/1 -> Mux/1
  Mux/1 -> RefVdVq/1

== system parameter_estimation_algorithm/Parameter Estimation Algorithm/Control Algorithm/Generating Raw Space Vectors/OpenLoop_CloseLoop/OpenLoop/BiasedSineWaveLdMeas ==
  Vd_ref : Inport
  Freq : Inport  Port=2
  Constant1 : Constant  Value=0  OutDataTypeStr=single  SampleTime=-1
  Mux : Mux  Inputs=2
  Sine2 : Subsystem
  RefVdVq : Outport  VectorParamsAs1DForOutWhenUnconnected=off
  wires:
  Constant1/1 -> Mux/2
  Sine2/1(sinBiased) -> Mux/1
  Mux/1 -> RefVdVq/1
  Freq/1 -> Sine2/1(Freq)
  Vd_ref/1 -> Sine2/2(Vd_ref)

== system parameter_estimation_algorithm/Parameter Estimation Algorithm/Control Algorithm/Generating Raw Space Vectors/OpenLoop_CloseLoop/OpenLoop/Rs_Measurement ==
  Vd_ref : Inport
  Mux1 : Mux  Inputs=2
  Vq_ref : Constant  Value=0  OutDataTypeStr=single  SampleTime=-1
  RefVdVq : Outport  VectorParamsAs1DForOutWhenUnconnected=off
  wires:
  Vq_ref/1 -> Mux1/2
  Vd_ref/1 -> Mux1/1
  Mux1/1 -> RefVdVq/1

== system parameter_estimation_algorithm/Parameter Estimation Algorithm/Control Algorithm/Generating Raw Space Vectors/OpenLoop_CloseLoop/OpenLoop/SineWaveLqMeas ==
  Vd_ref : Inport
  Freq : Inport  Port=2
  Mux : Mux  Inputs=2
  Sine3 : Subsystem
  RefVdVq : Outport  VectorParamsAs1DForOutWhenUnconnected=off
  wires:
  Mux/1 -> RefVdVq/1
  Vd_ref/1 -> Sine3/1(Vd_ref), Mux/1
  Freq/1 -> Sine3/2(Freq)
  Sine3/1(sinWave) -> Mux/2

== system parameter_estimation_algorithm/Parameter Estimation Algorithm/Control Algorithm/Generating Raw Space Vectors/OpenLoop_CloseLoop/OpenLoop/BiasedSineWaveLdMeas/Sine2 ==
  note: sinAmp_ac*sin(SineWaveArr))*Ld_measure+Sine_Vdc
  Freq : Inport
  Vd_ref : Inport  Port=2
  Discrete-Time Integrator2 : DiscreteIntegrator  ExternalReset=rising  SampleTime=-1  ICPrevOutput=DiscIntNeverNeededParam  ICPrevScaledInput=DiscIntNeverNeededParam
  Gain1 : Gain  Gain=0.5  RndMeth=Nearest
  Omega_x_Ts : Gain  Gain=1.5*Ts
  Product : Product
  Reset_Logic : Subsystem
  Sine-Cosine Lookup : mcbcontrolslib/Sine-Cosine Lookup  AngleInput=Per-unit  N_points=1024
  Sum : Sum  Inputs=|++
  Terminator : Terminator
  sinBiased : Outport  VectorParamsAs1DForOutWhenUnconnected=off
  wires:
  Discrete-Time Integrator2/1 -> Sine-Cosine Lookup/1, Reset_Logic/1(FeedBack)
  Vd_ref/1 -> Sum/2, Gain1/1
  Reset_Logic/1(Reset) -> Discrete-Time Integrator2/2
  Product/1 -> Sum/1
  Freq/1 -> Omega_x_Ts/1, Discrete-Time Integrator2/1
  Sum/1 -> sinBiased/1
  Omega_x_Ts/1 -> Reset_Logic/2(Omega*Ts)
  Sine-Cosine Lookup/1 -> Product/1
  Gain1/1 -> Product/2
  Sine-Cosine Lookup/2 -> Terminator/1

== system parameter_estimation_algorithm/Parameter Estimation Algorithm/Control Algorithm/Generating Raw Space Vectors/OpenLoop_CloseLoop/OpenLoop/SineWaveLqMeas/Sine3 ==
  note: sinAmp_ac*sin(SineWaveArr))*Ld_measure
  Vd_ref : Inport
  Freq : Inport  Port=2
  Discrete-Time Integrator2 : DiscreteIntegrator  ExternalReset=rising  SampleTime=-1  ICPrevOutput=DiscIntNeverNeededParam  ICPrevScaledInput=DiscIntNeverNeededParam
  Gain : Gain  Gain=0.5  RndMeth=Nearest
  Omega*Ts : Gain  Gain=1.5*Ts
  Product : Product
  Reset_Logic : Subsystem
  Sine-Cosine Lookup : mcbcontrolslib/Sine-Cosine Lookup  AngleInput=Per-unit  N_points=1024
  Terminator : Terminator
  sinWave : Outport  VectorParamsAs1DForOutWhenUnconnected=off
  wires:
  Sine-Cosine Lookup/1 -> Product/1
  Omega*Ts/1 -> Reset_Logic/2(Omega*Ts)
  Product/1 -> sinWave/1
  Freq/1 -> Discrete-Time Integrator2/1, Omega*Ts/1
  Gain/1 -> Product/2
  Reset_Logic/1(Reset) -> Discrete-Time Integrator2/2
  Discrete-Time Integrator2/1 -> Sine-Cosine Lookup/1, Reset_Logic/1(FeedBack)
  Vd_ref/1 -> Gain/1
  Sine-Cosine Lookup/2 -> Terminator/1
